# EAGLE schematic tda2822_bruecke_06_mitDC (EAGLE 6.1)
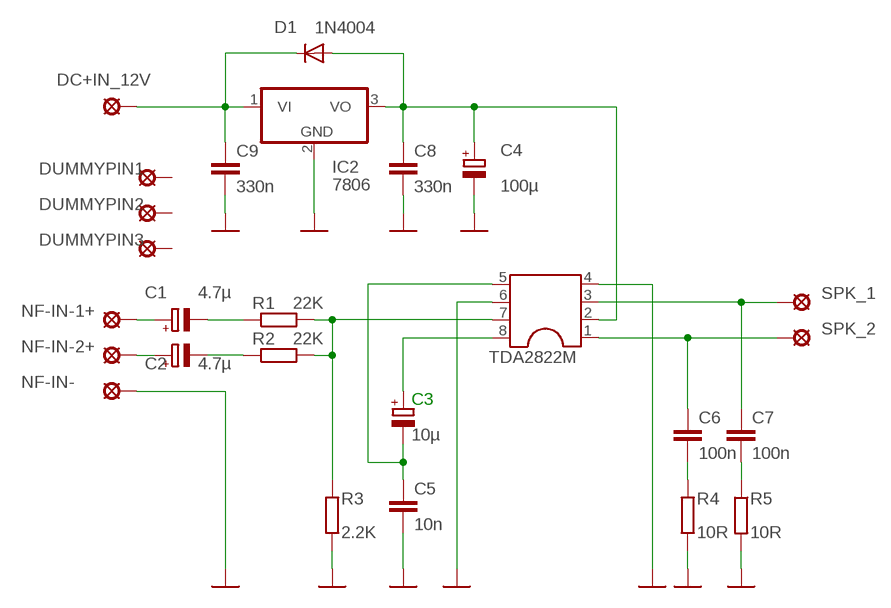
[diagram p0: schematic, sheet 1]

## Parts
C1  4.7µ  CPOL-EUE2.5-7  [E2,5-7]
C2  4.7µ  CPOL-EUE2.5-7  [E2,5-7]
C3  10µ  CPOL-EUE3.5-8  [E3,5-8]
C4  100µ  CPOL-EUE3.5-10  [E3,5-10]
C5  10n  C-EU050-024X044  [C050-024X044]
C6  100n  C-EU075-032X103  [C075-032X103]
C7  100n  C-EU075-032X103  [C075-032X103]
C8  330n  C-EU050-024X044  [C050-024X044]
C9  330n  C-EU050-024X044  [C050-024X044]
D1  1N4004  [DO41-10]
DC+IN_12V  LSP10  [LSP10]
DUMMYPIN1  LSP10  [LSP10]
DUMMYPIN2  LSP10  [LSP10]
DUMMYPIN3  LSP10  [LSP10]
IC2  7806  7805TV  [TO220V]
NF-IN-  LSP10  [LSP10]
NF-IN-1+  LSP10  [LSP10]
NF-IN-2+  LSP10  [LSP10]
R1  22K  R-EU_0207/7  [0207/7]
R2  22K  R-EU_0207/7  [0207/7]
R3  2.2K  R-EU_0207/7  [0207/7]
R4  10R  R-EU_0207/7  [0207/7]
R5  10R  R-EU_0207/7  [0207/7]
SPK_1  LSP10  [LSP10]
SPK_2  LSP10  [LSP10]
TDA2822M  DIL8  [DIL08]

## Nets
GND: C4.- C5.2 C8.2 C9.2 IC2.2(GND) NF-IN-.MP R3.1 R4.1 R5.2 TDA2822M.4 TDA2822M.6
N$1: R1.2 R2.2 R3.2 TDA2822M.7
N$2: C3.- C5.1 TDA2822M.5
N$3: C3.+ TDA2822M.8
N$4: C9.1 D1.C DC+IN_12V.MP IC2.1(VI)
N$5: C4.+ C8.1 D1.A IC2.3(VO) TDA2822M.2
N$6: C7.1 SPK_1.MP TDA2822M.3
N$7: C7.2 R5.1
N$8: C1.+ NF-IN-1+.MP
N$9: C6.1 SPK_2.MP TDA2822M.1
N$10: C6.2 R4.2
N$11: C2.- R2.1
N$12: C1.- R1.1
N$13: C2.+ NF-IN-2+.MP
Unconnected: DUMMYPIN1.MP DUMMYPIN2.MP DUMMYPIN3.MP

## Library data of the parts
C1-C4 = rcl:CPOL-EU: POLARIZED CAPACITOR, European symbol
C5-C9 = rcl:C-EU: CAPACITOR, European symbol
D1 = diode:1N4004: DIODE
DC+IN_12V DUMMYPIN1-DUMMYPIN3 NF-IN- NF-IN-1+ NF-IN-2+ SPK_1 SPK_2 = solpad:LSP10: SOLDER PAD
IC2 = linear:78*: Positive VOLTAGE REGULATOR Source: http://cache.national.com/ds/LM/LM78L05.pdf http://www.fairchildsemi.com/ds/LM/LM7805.pdf
R1-R5 = rcl:R-EU_: RESISTOR, European symbol
TDA2822M = ic-package:DIL8: Dual In Line / Socket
